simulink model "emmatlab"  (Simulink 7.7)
settings: Solver=FixedStepDiscrete  StartTime=0.0  StopTime=100  FixedStep=0.1  RelTol=1e-3
libraries: simulink x2

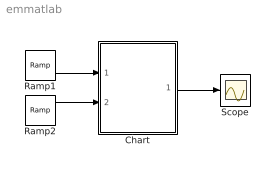
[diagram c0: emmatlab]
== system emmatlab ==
  Chart : Stateflow chart  TreatAsAtomicUnit=on
  Ramp1 : simulink/Sources/Ramp  SystemSampleTime=-1  slope=1  start=0  X0=0
  Ramp2 : simulink/Sources/Ramp  SystemSampleTime=-1  slope=2  start=25  X0=0
  Scope : Scope
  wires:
  Ramp1/1 -> Chart/1(in1)
  Ramp2/1 -> Chart/2(in2)
  Chart/1(out) -> Scope/1

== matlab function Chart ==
function y=minimum(x1,x2)
% Die Funktion minimum(x) erwartet als Eingabe 
% einen Vektor der Dimension 2 bestehend aus 
% double-Werten. Als Rückgabewert y wird das Minimum 
% der beiden Werte geliefert.
if x1>x2
    y=x2;
else
    y=x1;
end
